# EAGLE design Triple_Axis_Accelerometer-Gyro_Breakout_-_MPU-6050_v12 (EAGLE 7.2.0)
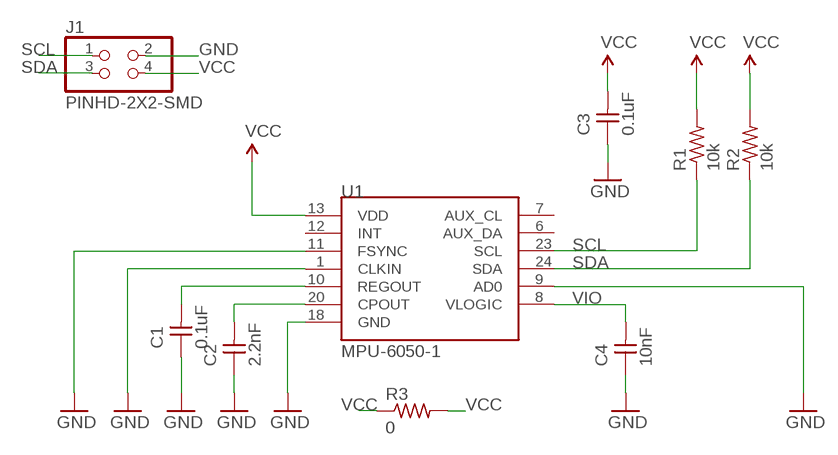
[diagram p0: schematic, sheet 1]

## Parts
C1  0.1uF  UNPOLARIZED_CAPACITOR1206  [1206]
C2  2.2nF  UNPOLARIZED_CAPACITOR1206  [1206]
C3  0.1uF  UNPOLARIZED_CAPACITOR1206  [1206]
C4  10nF  UNPOLARIZED_CAPACITOR1206  [1206]
J1  PINHD-2X2-SMD  [2X02SMD]
R1  10k  RESISTOR1206  [1206]
R2  10k  RESISTOR1206  [1206]
R3  0  RESISTOR1206  [1206]
U1  MPU-6050-1  [QFN-24-4MM2]

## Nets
CLKIN: U1.1(CLKIN)
FSYNC: U1.11(FSYNC)
GND: C1.1 C2.1 C3.1 C4.1 J1.2 U1.9(AD0) U1.18(GND)
N$3: C2.2 U1.20(CPOUT)
N$5: C1.2 U1.10(REGOUT)
SCL: J1.1 R1.1 U1.23(SCL)
SDA: J1.3 R2.1 U1.24(SDA)
VCC: C3.2 J1.4 R1.2 R2.2 R3.1 R3.2 U1.13(VDD)
VIO: C4.2 U1.8(VLOGIC)
Unconnected: U1.6(AUX_DA) U1.7(AUX_CL) U1.12(INT)

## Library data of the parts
C1-C4 = ng:UNPOLARIZED_CAPACITOR: unpolarized_capacitor
J1 = fab:PINHD-2X2-SMD
R1-R3 = ng:RESISTOR
U1 = Testing:MPU-6050

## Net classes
0 Default: width 0.203 mm
1 vcc: width 0.254 mm
2 GND: width 0.813 mm

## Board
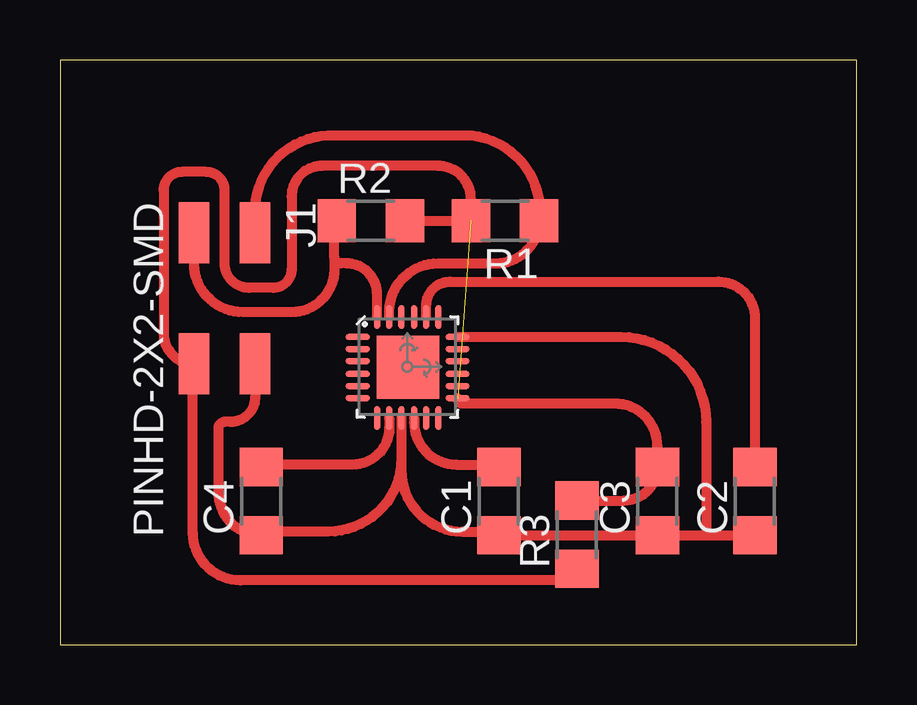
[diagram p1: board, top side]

Size 33.2 x 24.37 mm. Coordinates in mm from the lower left corner, seen from the top.
Outline: 0,0 33.2,0 33.2,24.37 0,24.37 0,0
Copper layers (1*16): Top 0.035mm / dielectric 1.5mm / Bottom 0.035mm
Design rules "default": minimum track width 10mil, minimum drill 24mil, track to track 8mil, track to pad 8mil, pad to pad 8mil, via to via 8mil, smd to smd 8mil, copper to edge 40mil, drill to drill 8mil, minimum pad ring 10mil, minimum via ring 8mil, stop-mask expansion 4mil, vias tented up to drill 0mil, thermal gap 10mil

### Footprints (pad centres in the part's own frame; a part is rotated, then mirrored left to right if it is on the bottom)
1206 = smd 1.6 x 1.803: 1 -1.422,0; 2 1.422,0
2X02SMD = smd 2.54 x 1.27: 1 -2.54,1.27; 2 2.92,1.27; 3 -2.54,-1.27; 4 2.92,-1.27
QFN-24-4MM2 = smd 1.016 x 0.254: 1 -2.066,1.257; 2 -2.066,0.75; 3 -2.066,0.247; 4 -2.066,-0.287; 5 -2.066,-0.792; 6 -2.066,-1.297; 13 2.086,-1.297; 14 2.086,-0.792; 15 2.086,-0.287; 16 2.086,0.247; 17 2.086,0.75; 18 2.086,1.257 | smd 0.254 x 1.016: 7 -1.267,-2.122; 8 -0.762,-2.122; 9 -0.258,-2.122; 10 0.278,-2.122; 11 0.78,-2.122; 12 1.287,-2.122; 19 1.287,2.082; 20 0.78,2.082; 21 0.278,2.082; 22 -0.258,2.082; 23 -0.762,2.082; 24 -1.267,2.082 | smd 2.616 x 2.616: P$1 0.02,-0.01

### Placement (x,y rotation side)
C1  18.29,5.99 90 top
C2  28.96,5.99 90 top
C3  24.89,5.99 90 top
C4  8.38,5.99 90 top
J1  6.86,14.63 270 top
R1  18.54,17.68 180 top
R2  12.95,17.68 0 top
R3  21.54,4.6 90 top
U1  14.48,11.58 0 top

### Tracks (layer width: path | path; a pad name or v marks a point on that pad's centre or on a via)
GND
  Top 0.406: U1.9 14.22,7.77 | 14.22,7.77 arc-90 11.18,4.72 8.53,4.72 arc90 C4.1 arc-90 6.6,6.35 6.6,9.04 arc-90 6.86,9.3 7.11,9.3 arc90 8.13,10.31 J1.2 | 14.22,7.77 14.22,7.27 arc90 16.76,4.72 18.64,4.72 arc-90 18.8,4.57 | C1.1 18.8,4.57 | 18.8,4.57 C3.1 26.92,4.57 | 26.92,4.57 C2.1 | 26.92,4.57 26.92,9.3 arc90 23.38,12.84 U1.18
N$3
  Top 0.406: U1.20 15.26,14.14 arc-90 16.26,15.14 27.43,15.14 arc-90 28.96,13.61 C2.2
N$5
  Top 0.406: U1.10 14.76,9.27 arc90 16.51,7.52 18.19,7.52 arc-90 C1.2
SCL
  Top 0.406: U1.23 13.72,13.87 arc-90 15.75,15.9 18.19,15.9 arc90 R1.1 arc90 17.17,21.23 11.18,21.23 arc90 8.13,17.93 J1.1
SDA
  Top 0.406: U1.24 13.21,14.63 arc90 11.94,15.9 11.68,15.9 arc-90 11.43,16.15 | 11.43,16.15 11.43,17.58 arc-90 R2.1 | 11.43,16.15 11.43,15.65 arc-90 9.65,13.87 7.62,13.87 arc-90 5.59,15.9 J1.3
VCC  (1 unrouted)
  Top 0.406: R2.2 R1.2 17.12,18.59 arc90 15.75,19.96 10.92,19.96 arc90 9.65,18.69 9.65,15.65 arc-90 8.89,14.88 7.87,14.88 arc-90 6.86,15.9 6.86,18.95 arc90 6.1,19.71 5.08,19.71 arc90 4.32,18.95 4.32,12.98 arc90 J1.4 arc90 5.54,11.66 5.54,4.67 arc90 7.52,2.69 21.13,2.69 arc90 21.54,3.1 R3.1 | U1.13 arc90 16.79,10.06 23.11,10.06 arc-90 24.89,8.28 C3.2 arc-90 23.5,6.02 R3.2
VIO
  Top 0.406: U1.8 13.72,9.04 arc-90 12.19,7.52 8.48,7.52 arc90 C4.2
